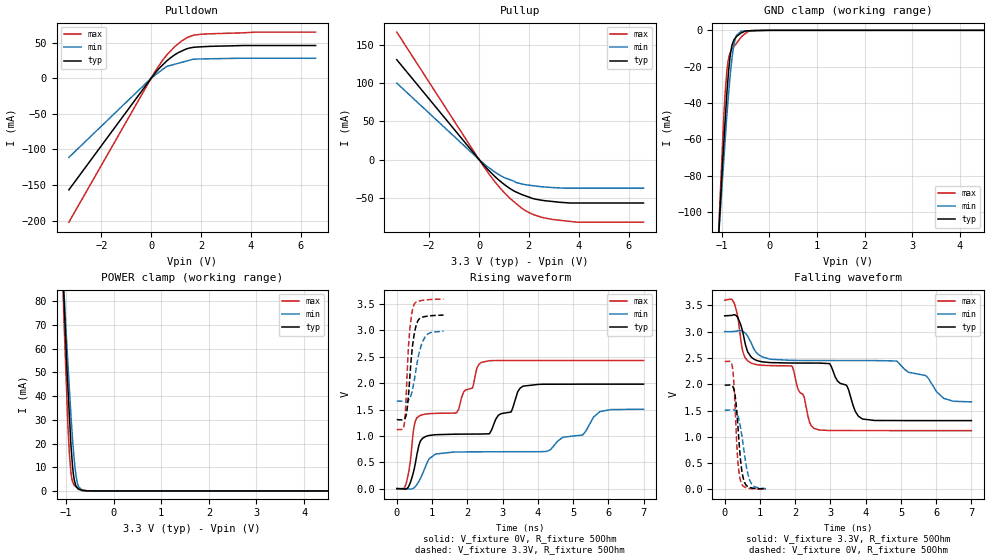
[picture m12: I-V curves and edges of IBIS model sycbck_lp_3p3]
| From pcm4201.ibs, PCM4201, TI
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|   sycbck_lp_3p3 Model
[Model]   sycbck_lp_3p3
Model_type   I/O
Polarity   Non-Inverting
Enable   Active-Low
Vinl = 0.99
Vinh = 2.31
Vmeas = 1.65
Vref = 1.65
Cref = 2pF
Rref = 50
|   typ   min   max
|   (nom PVT)   (fast PVT)   (slow PVT)
|C_comp from frequency sweep method (F=6.94MHz)
|Average
C_comp   1.202e-12   1.069e-12   1.381e-12
|ON state : BUFFER OUTPUT TURNED HIGH
|C_comp   1.247e-12   1.127e-12   1.445e-12
|OFF state: BUFFER IN HIGH IMPEDANCE
|C_comp   1.157e-12   1.010e-12   1.317e-12
|C_comp from LC tank measurement(L=1nH)
|Average
|Resonant Frequency(Hz)   7.760e+09   7.900e+09   7.500e+09
|C_comp   4.211e-13   4.066e-13   4.508e-13
|ON state : BUFFER OUTPUT TURNED HIGH
|Resonant Frequency(Hz)   7.720e+09   7.770e+09   7.500e+09
|C_comp   4.254e-13   4.200e-13   4.508e-13
|OFF state: BUFFER IN HIGH IMPEDANCE
|Resonant Frequency(Hz)   7.800e+09   8.030e+09   7.500e+09
|C_comp   4.168e-13   3.932e-13   4.508e-13
| Where nom  PVT is Nominal Process, 3.3V, 35C
|   Fast PVT is Strong Process,  3.6V, -10C
|   Slow PVT is Weak Process,   3V, 80C
[Model Spec]
Vinl   0.99   0.9   1.08
Vinh   2.31   2.1   2.52
[Voltage Range]   3.3   3   3.6
|Ambient Temperature   25   70   -10
|Junction Temperature
[Temperature Range]   35   80   -10
[Pullup Reference]   3.3   3   3.6
[Pulldown Reference]   0   0   0
[Power Clamp Reference]   3.3   3   3.6
[GND Clamp Reference]   0   0   0
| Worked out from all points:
|   slope of the pulldown table from 0 to 0.495 V, typ, clamps not added: 25 ohm
|   slope of the pullup table from 0 to 0.495 V, typ, clamps not added: 28.1 ohm
|   GND clamp passes 1 mA (typ) near -0.56 V on its own axis
|   POWER clamp passes 1 mA (typ) near -0.75 V on its own axis
|   falling waveform, V_fixture 3.3V, R_fixture 50Ohm: 20-80 % time 3.05ns typ, 5.16ns min, 1.89ns max; typ from 3.3 V to 1.31 V
|   rising waveform, V_fixture 0V, R_fixture 50Ohm: 20-80 % time 2.81ns typ, 4.71ns min, 1.78ns max; typ from 0 V to 1.98 V
|   rising waveform, V_fixture 3.3V, R_fixture 50Ohm: 20-80 % time 163ps typ, 235ps min, 127ps max; typ from 1.31 V to 3.29 V
|   falling waveform, V_fixture 0V, R_fixture 50Ohm: 20-80 % time 148ps typ, 212ps min, 113ps max; typ from 1.98 V to 0.008 V
[Pulldown]
|   Voltage   I(typ)   I(min)   I(max)
-3.3V     -156.9mA   -111.3mA   -202.4mA
18mV      811.1uA    603.1uA    1.128mA
172.8mV   7.787mA    4.701mA    10.34mA
633mV     24.59mA    16.74mA    32.89mA
939.6mV   32.82mA    19.66mA    44.25mA
1.246V    38.58mA    22.58mA    52.93mA
1.469V    41.87mA    24.7mA     57.59mA
1.692V    43.49mA    26.82mA    60.46mA
2.012V    44.26mA    27.15mA    61.95mA
4.208V    46.06mA    28.16mA    64.93mA
6.6V      46.06mA    28.16mA    64.97mA
[GND Clamp]
|   Voltage   I(typ)   I(min)   I(max)
-3.3V     -1.347A    -1.084A    -1.74A
-1.105V   -131.4mA   -127.7mA   -135mA
-1.051V   -104.8mA   -106.8mA   -100.1mA
-957.6mV  -60.85mA   -70.73mA   -46.53mA
-928.8mV  -48.57mA   -59.64mA   -33.58mA
-874.8mV  -27.6mA    -40.04mA   -17.83mA
-821.7mV  -13.1mA    -23.71mA   -12.19mA
-747mV    -5.242mA   -7.776mA   -8.933mA
-693mV    -3.387mA   -2.784mA   -7.073mA
-594mV    -1.406mA   -492.9uA   -3.663mA
-133.2mV  -88.06uA   -151.6nA   -18.24nA
6.6V      0A         0A         0A
[Pullup]
|   Voltage   I(typ)   I(min)   I(max)
-3.3V     130.7mA    100.1mA    166.9mA
172.8mV   -6.598mA   -4.879mA   -8.507mA
633mV     -22.16mA   -16.42mA   -28.97mA
939.6mV   -30.84mA   -22.42mA   -40.79mA
1.399V    -41.23mA   -28.32mA   -55.25mA
1.492V    -42.61mA   -30.16mA   -57.77mA
1.706V    -45.8mA    -31.93mA   -63.61mA
2.167V    -51.22mA   -34.33mA   -71.98mA
2.934V    -54.99mA   -36.73mA   -78.49mA
3.935V    -56.99mA   -37.53mA   -82.14mA
6.6V      -56.99mA   -37.53mA   -82.14mA
[POWER Clamp]
|   Voltage   I(typ)   I(min)   I(max)
-3.3V     1.329A     1.069A     1.72A
-1.086V   100.9mA    100.9mA    99.43mA
-1.044V   81.27mA    84.53mA    72.38mA
-961.2mV  43.68mA    53.95mA    27.77mA
-928.8mV  31.31mA    42.74mA    15.35mA
-896.4mV  19.07mA    31.56mA    7.563mA
-864.6mV  10.62mA    22.16mA    3.994mA
-831.6mV  5.062mA    13.97mA    2.491mA
-789mV    1.968mA    6.21mA     1.731mA
-745.8mV  785.2uA    2.283mA    1.149mA
-591mV    80.73uA    40.26uA    223.7uA
6.6V      0A         0A         0A
[Ramp]
R_load = 50
|   typ   min   max
dV/dt_r   1.18901/2.81103e-09   0.903979/4.70574e-09   1.45875/1.78614e-09
dV/dt_f   1.19482/3.05129e-09   0.801605/5.15319e-09   1.48886/1.88926e-09
[Falling Waveform]
V_fixture = 3.3V
V_fixture_min = 3V
V_fixture_max = 3.6V
R_fixture = 50Ohm
|   Time   V(typ)   V(min)   V(max)
0s        3.3V       3V         3.6V
269ps     3.321V     3.003V     3.543V
644ps     2.629V     2.921V     2.451V
1.07ns    2.425V     2.518V     2.36V
1.916ns   2.403V     2.453V     2.338V
2.528ns   2.402V     2.451V     1.161V
2.978ns   2.388V     2.45V      1.12V
3.914ns   1.338V     2.45V      1.119V
4.874ns   1.31V      2.441V     1.118V
6.998ns   1.308V     1.664V     1.118V
[Rising Waveform]
V_fixture = 0V
V_fixture_min = 0V
V_fixture_max = 0V
R_fixture = 50Ohm
|   Time   V(typ)   V(min)   V(max)
0s        117uV      80.69uV    163.6uV
269ps     -8.106mV   -792.2uV   105.2mV
566ps     626.9mV    73.34mV    1.337V
920ps     1.009V     566.4mV    1.422V
1.691ns   1.033V     694mV      1.435V
2.393ns   1.035V     698mV      2.393V
3.584ns   1.944V     699.9mV    2.431V
5.27ns    1.981V     1.016V     2.431V
5.768ns   1.982V     1.462V     2.431V
6.998ns   1.982V     1.507V     2.431V
[Rising Waveform]
V_fixture = 3.3V
V_fixture_min = 3V
V_fixture_max = 3.6V
R_fixture = 50Ohm
|   Time   V(typ)   V(min)   V(max)
0s        1.309V     1.661V     1.119V
215ps     1.318V     1.65V      1.237V
245ps     1.349V     1.648V     1.476V
296ps     1.519V     1.656V     2.213V
344ps     1.872V     1.686V     2.813V
413ps     2.488V     1.79V      3.265V
479ps     2.864V     1.987V     3.474V
596ps     3.18V      2.455V     3.55V
809ps     3.266V     2.884V     3.579V
1.325ns   3.293V     2.987V     3.596V
[Falling Waveform]
V_fixture = 0V
V_fixture_min = 0V
V_fixture_max = 0V
R_fixture = 50Ohm
|   Time   V(typ)   V(min)   V(max)
0s        1.982V     1.508V     2.431V
167ps     1.987V     1.512V     2.428V
224ps     1.963V     1.515V     2.304V
257ps     1.914V     1.512V     2.057V
296ps     1.783V     1.496V     1.555V
368ps     1.262V     1.41V      585.4mV
464ps     468.2mV    1.118V     133.8mV
560ps     141.1mV    671.3mV    47.16mV
713ps     38.8mV     172.8mV    19.11mV
1.169ns   8.178mV    14.03mV    5.627mV
